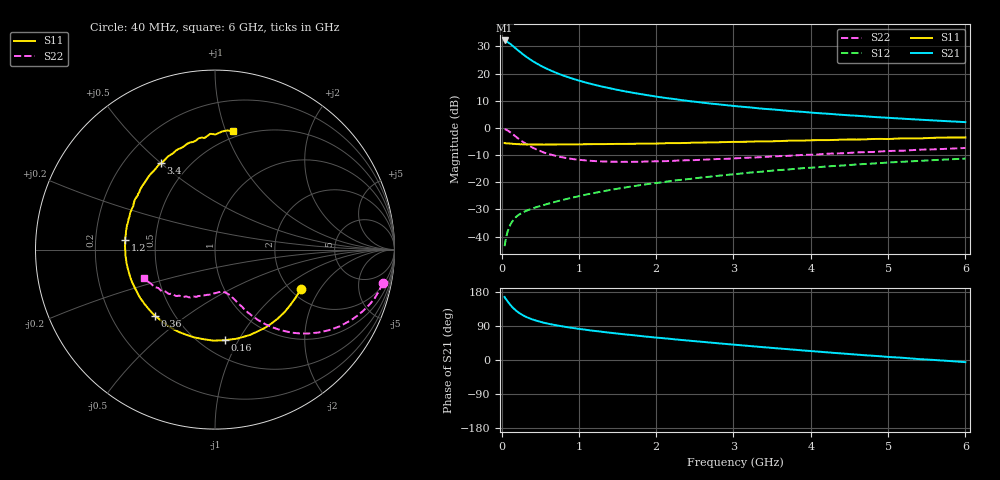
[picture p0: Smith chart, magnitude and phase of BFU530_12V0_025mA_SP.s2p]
! Filename:  P:\Prog\Test\Noise\ATS_data\Testdata_Net\03 Spar\BFU530_APG2013_40_A05_12p0V_025mA_SP_CM01_D.s2p
! Date/Time: Fri 26/Apr/2013 13:03:11
! BFU530_APG2013_40_A05_12p0V_1to25mA_SP_CM01_Bias8_R.s2p
! MDIF S-parameter v. bias file
! BFU530_APG2013_40_A05_12p0V_1to25mA_SP_CM01
! Date/time Wed Apr 24 20:41:12 2013
! VAR V_out= 12.0010
! VAR I_out= 24.9950
! VAR V_in= 0.7769
! VAR I_in= 0.2446
! Device data file deembeded for feedlines and parallel
! Original file: \03 Spar\BFU530_APG2013_40_A05_12p0V_025mA_SP_CM01_R.s2p
! Feed-files: PR047V01_250413_Feed1.s2p, PR047V01_250413_Feed2.s2p
! Parallel-file: PR047V01_250413_Par.s2p
# MHz S MA R 50
!  Freq-MHz  S11-mag  S11-arg  S21-mag  S21-arg  S12-mag  S12-arg  S22-mag  S22-arg
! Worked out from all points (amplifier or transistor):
!   98 points, 40 MHz to 6 GHz, reference 50 ohm
!   highest |S21| = 32.2 dB at 40 MHz (marker M1)
!   |S21| within 3 dB of that: start of sweep to 186.6 MHz
!   unconditionally stable (mu >= 1): 1.301 GHz to 3.548 GHz
!   at 300 MHz: K = 0.49, MSG = 28.7 dB, |S12| = -30.7 dB
!   at 1.6 GHz: K = 1.03, MAG = 16.6 dB, |S12| = -21.9 dB
!   at 6 GHz: K = 0.87, MSG = 6.7 dB, |S12| = -11.3 dB
!   S11 on the Smith chart (normalised r, x): 40 MHz: 2.27, -1.37; 160 MHz: 0.65, -0.88; 360 MHz: 0.39, -0.39; 1.2 GHz: 0.33, +0.05; 3.4 GHz: 0.35, +0.50; 6 GHz: 0.45, +1.06
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40  0.527 -24.4  40.76 166.3  0.006671 79.6  0.9532 -11.4
50  0.5232 -30.6  40.46 162.6  0.008171 77.6  0.9419 -14.3
90  0.5183 -52.7  37.12 151.6  0.01375 70.2  0.8756 -24.8
120  0.5141 -67.5  34.62 144.0  0.01719 65.5  0.8167 -31.5
140  0.5112 -76.1  32.82 139.5  0.01913 62.9  0.7766 -35.4
160  0.5079 -83.9  31.03 135.5  0.0209 60.7  0.7384 -38.7
200  0.5032 -97.5  27.79 128.4  0.02378 57.4  0.6657 -44.5
240  0.5009 -108.7  24.98 122.6  0.02612 55.2  0.6036 -49.1
300  0.4988 -121.9  21.47 115.6  0.02901 53.2  0.5281 -54.2
360  0.498 -132.1  18.68 110.2  0.03146 52.4  0.4695 -58.0
460  0.4956 -144.7  15.22 103.2  0.03518 52.5  0.3984 -62.2
600  0.4957 -157.2  12.05 95.9  0.04026 53.8  0.3349 -66.0
800  0.4977 -169.3  9.214 88.3  0.04769 55.8  0.2859 -69.9
1050  0.5008 179.3  7.109 80.8  0.0575 57.6  0.2558 -74.1
1200  0.5033 173.9  6.244 76.8  0.06355 58.2  0.2462 -76.5
1600  0.5093 161.6  4.709 67.5  0.08022 58.6  0.2382 -83.3
2050  0.5194 151.0  3.684 58.3  0.09898 57.6  0.244 -91.5
3100  0.5556 128.1  2.463 38.9  0.1451 52.7  0.2799 -110.8
3400  0.569 122.0  2.245 33.6  0.1583 50.6  0.2926 -116.3
4100  0.5964 109.8  1.872 22.1  0.1899 45.5  0.3257 -128.1
5200  0.6457 92.4  1.478 5.7  0.2392 36.4  0.3819 -145.9
6000  0.6677 81.2  1.28 -5.6  0.2727 28.9  0.4281 -158.3
